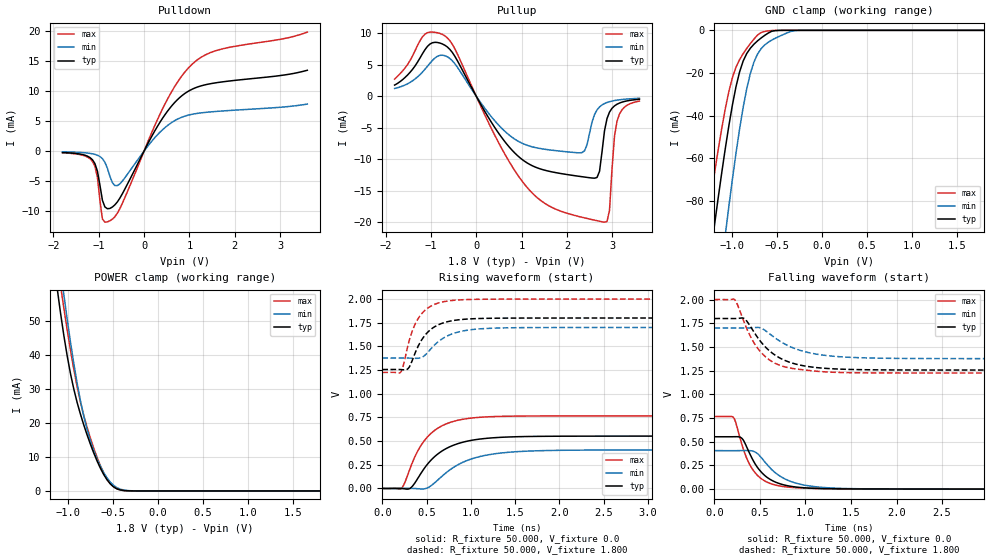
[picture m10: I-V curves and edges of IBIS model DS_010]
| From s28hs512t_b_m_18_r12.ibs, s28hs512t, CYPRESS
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|   Model DS_010
[Model] DS_010
Model_type 3-state
Polarity   Non-Inverting
Enable   Active-High
Vmeas =  0.900V
Cref =  15.000pF
C_comp   5.334pF   5.23pF   5.767pF
[Temperature Range]   25.000   0.125k   -40.000
[Voltage Range]   1.800V   1.700V   2.000V
[Pullup Reference]   1.800V   1.700V   2.000V
[Pulldown Reference]   0.0V   0.0V   0.0V
[POWER Clamp Reference]   1.800V   1.700V   2.000V
[GND Clamp Reference]   0.0V   0.0V   0.0V
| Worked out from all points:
|   slope of the pulldown table from 0 to 0.27 V, typ, clamps not added: 70.9 ohm
|   slope of the pullup table from 0 to 0.27 V, typ, clamps not added: 79.8 ohm
|   GND clamp passes 1 mA (typ) near -0.59 V on its own axis
|   POWER clamp passes 1 mA (typ) near -0.48 V on its own axis
|   rising waveform, R_fixture 50.000, V_fixture 0.0: 20-80 % time 364ps typ, 435ps min, 300ps max; typ from 0 V to 0.553 V
|   rising waveform, R_fixture 50.000, V_fixture 1.800: 20-80 % time 221ps typ, 281ps min, 186ps max; typ from 1.26 V to 1.8 V
|   falling waveform, R_fixture 50.000, V_fixture 0.0: 20-80 % time 244ps typ, 317ps min, 205ps max; typ from 0.553 V to 0 V
|   falling waveform, R_fixture 50.000, V_fixture 1.800: 20-80 % time 346ps typ, 420ps min, 288ps max; typ from 1.8 V to 1.26 V
[Pulldown]
|Voltage   I(typ)   I(min)   I(max)
-1.8V     -252.5uA   -134uA     -302.8uA
-1.14V    -1.461mA   -464.4uA   -1.736mA
-1.03V    -3.372mA   -704.8uA   -4.413mA
-920mV    -8.226mA   -1.27mA    -11.35mA
-755mV    -9.59mA    -4.228mA   -11.66mA
-645mV    -8.995mA   -5.77mA    -10.98mA
-535mV    -7.872mA   -5.49mA    -9.628mA
400mV     5.394mA    3.504mA    6.944mA
730mV     8.539mA    5.3mA      11.43mA
1.06V     10.33mA    6.136mA    14.5mA
1.665V    11.48mA    6.65mA     16.93mA
3.6V      13.49mA    7.838mA    19.86mA
[Pullup]
|Voltage   I(typ)   I(min)   I(max)
-1.8V     1.752mA    1.214mA    2.694mA
-1.13V    7.359mA    4.261mA    9.823mA
-690mV    8.057mA    6.408mA    9.538mA
520mV     -6.128mA   -4.777mA   -7.72mA
1.18V     -10.81mA   -7.913mA   -14.92mA
2.335V    -12.76mA   -8.934mA   -19.19mA
2.665V    -12.87mA   -2.175mA   -19.72mA
2.83V     -5.479mA   -1.168mA   -19.96mA
2.94V     -2.526mA   -877.2uA   -18.1mA
3.05V     -1.543mA   -698.5uA   -6.371mA
3.105V    -1.281mA   -633.1uA   -4.001mA
3.6V      -491.8uA   -340uA     -786.1uA
[GND_clamp]
|Voltage   I(typ)   I(min)   I(max)
-1.8V     -294mA     -373mA     -247.3mA
-1.28V    -116.8mA   -168.5mA   -89.46mA
-1.2V     -91.34mA   -138.7mA   -67.04mA
-1.08V    -55.6mA    -96.11mA   -36.91mA
-1.04V    -44.83mA   -82.66mA   -28.74mA
-1V       -34.98mA   -69.76mA   -22.14mA
-920mV    -19.48mA   -46.23mA   -13.73mA
-800mV    -8.377mA   -20.18mA   -6.205mA
-680mV    -3.579mA   -8.59mA    -1.029mA
-560mV    -408.3uA   -4.544mA   -113.8uA
-280mV    -162.8nA   -73.51uA   -82.13nA
1.8V      272.8pA    325nA      188.3pA
[POWER_clamp]
|Voltage   I(typ)   I(min)   I(max)
-1.8V     236.7mA    239.1mA    251.1mA
-1.123V   59.68mA    73.25mA    67.66mA
-1.086V   52.46mA    65.42mA    60.6mA
-1.049V   45.83mA    57.89mA    53.9mA
-938mV    30.03mA    37.57mA    35.87mA
-864mV    22.62mA    26.6mA     26.18mA
-790mV    16.52mA    18.14mA    18.76mA
-716mV    11.21mA    11.92mA    12.63mA
-642mV    6.708mA    7.258mA    7.47mA
-494mV    1.178mA    1.619mA    1.205mA
-272mV    6.291uA    28.11uA    4.439uA
1.8V      0A         0A         0A
[Ramp]
| variable   typ   min   max
dV/dt_r   0.332/0.363n   0.244/0.435n   0.460/0.300n
dV/dt_f   0.326/0.346n   0.194/0.419n   0.465/0.288n
R_load = 50.000
[Rising Waveform]
R_fixture= 50.000
V_fixture= 0.0
V_fixture_min= 0.0
V_fixture_max= 0.0
|time   V(typ)   V(min)   V(max)
0s        3.294uV    4.239uV    3.653uV
218ps     153.1uV    413.9uV    3.161mV
330ps     14.08mV    726.9uV    252.7mV
440ps     165.3mV    -5.692mV   460.2mV
570ps     318.3mV    43.56mV    598.2mV
751ps     435.6mV    188.3mV    692.6mV
971ps     501.9mV    300.4mV    739.5mV
1.341ns   540.1mV    374.5mV    761.3mV
1.861ns   550.9mV    400.6mV    765.7mV
6ns       552.8mV    406.4mV    766.3mV
[Rising Waveform]
R_fixture= 50.000
V_fixture= 1.800
V_fixture_min= 1.700
V_fixture_max= 2.000
|time   V(typ)   V(min)   V(max)
0s        1.256V     1.377V     1.225V
205ps     1.256V     1.377V     1.226V
232ps     1.254V     1.377V     1.282V
297ps     1.273V     1.377V     1.537V
345ps     1.37V      1.375V     1.68V
414ps     1.519V     1.376V     1.808V
564ps     1.691V     1.491V     1.933V
754ps     1.765V     1.619V     1.981V
1.337ns   1.798V     1.695V     1.999V
6ns       1.8V       1.7V       2V
[Falling Waveform]
R_fixture= 50.000
V_fixture= 0.0
V_fixture_min= 0.0
V_fixture_max= 0.0
|time   V(typ)   V(min)   V(max)
0s        552.8mV    406.3mV    766.4mV
207ps     553mV      406.2mV    758.4mV
304ps     533.6mV    406.9mV    463.2mV
360ps     432.9mV    407.6mV    313.8mV
430ps     294.7mV    398.4mV    194.1mV
575ps     126.8mV    263.4mV    75.5mV
756ps     46.67mV    116.9mV    27.7mV
1.046ns   11.04mV    33.32mV    9.051mV
1.456ns   3.075mV    6.339mV    2.539mV
6ns       5.324uV    28.6uV     -2.51uV
[Falling Waveform]
R_fixture= 50.000
V_fixture= 1.800
V_fixture_min= 1.700
V_fixture_max= 2.000
|time   V(typ)   V(min)   V(max)
0s        1.8V       1.7V       2V
217ps     1.799V     1.7V       2.002V
335ps     1.794V     1.699V     1.74V
415ps     1.686V     1.702V     1.575V
509ps     1.555V     1.7V       1.446V
679ps     1.406V     1.586V     1.322V
899ps     1.318V     1.477V     1.268V
1.179ns   1.277V     1.416V     1.239V
1.684ns   1.259V     1.384V     1.227V
6ns       1.256V     1.377V     1.225V
